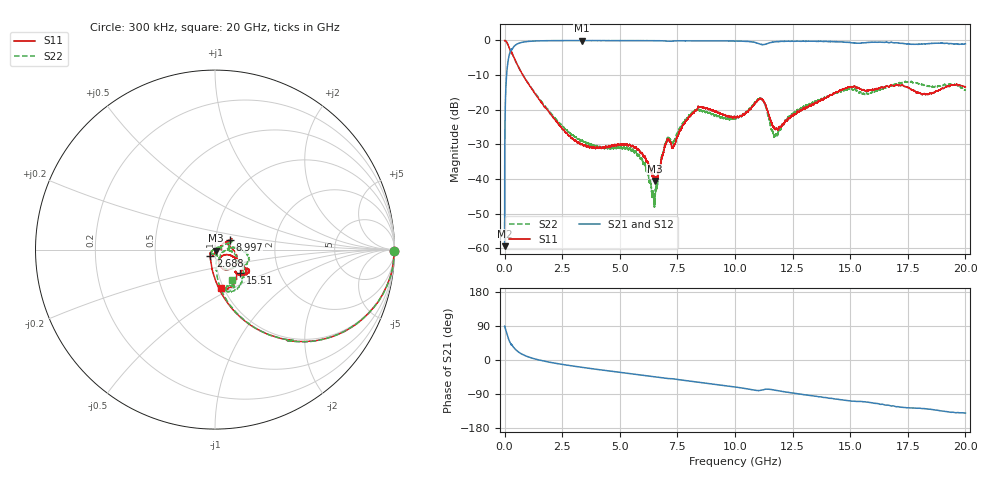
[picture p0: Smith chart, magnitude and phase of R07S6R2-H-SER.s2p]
!{R07S6R2}
!Johanson Technology Inc.
!www.johansontechnology.com
!Test Board Conditions:
!Substrate Type  RO4350B
!Substrate Thickness  10 mil
!Substrate Dk  3.66
!TL Type: GCPW
!TL Trace Width  21 mil
!TL Gap  20 mil
!Electrode orientation  Horizontal
!DUT TOPOLOGY	SERIES
!Mounting Pad LxW  16x21 mil
! Created Sat Feb  6 11:37:33 2021
# hz S ma R 50
! 2 Port Network Data from SP1.SP block
! freq  magS11  angS11  magS21  angS21  magS12  angS12  magS22  angS22
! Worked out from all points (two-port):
!   20001 points, 300 kHz to 20 GHz, reference 50 ohm
!   highest |S21| = -0.03 dB at 3.357 GHz (marker M1); lowest = -59.4 dB at 300 kHz (marker M2)
!   |S21| within 3 dB of the highest: 257.6 MHz to end of sweep
!   lowest |S11| = -40.5 dB at 6.525 GHz (marker M3), VSWR 1.02, Z = 50.7 - j0.674 ohm
!   |S11| at or under -10 dB: 794.4 MHz to end of sweep
!   |S22| runs from -48.2 to 0.0 dB; largest |S21 - S12| = 0.012
!   S11 on the Smith chart (normalised r, x): 300 kHz: open; 2.688 GHz: 0.95, -0.07; 8.997 GHz: 1.17, +0.13; 15.51 GHz: 1.28, -0.35; 20 GHz: 0.97, -0.43
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300000  0.9982 -0.4  0.001074 89.1  0.001152 93.4  0.9994 -0.4
1.093e8  0.919 -23.7  0.3903 66.6  0.3907 66.6  0.919 -23.6
2.833e8  0.6659 -49.9  0.7374 40.8  0.7376 40.7  0.6686 -49.8
9.053e8  0.2741 -79.2  0.9581 11.1  0.9587 11.1  0.2772 -77.8
2.6883e9  0.04622 -125.2  0.9949 -13.3  0.9957 -13.4  0.05084 -77.8
3.3343e9  0.0319 -144.2  0.9953 -19.1  0.996 -19.1  0.03585 -69.2
3.3573e9  0.03183 -144.9  0.9968 -19.3  0.9959 -19.3  0.036 -69.0
5.6323e9  0.0282 -109.2  0.9925 -37.5  0.9935 -37.5  0.02409 -141.8
6.5253e9  0.009416 -44.9  0.9919 -44.6  0.9918 -44.6  0.005167 92.2
6.6673e9  0.01203 -5.2  0.9913 -45.7  0.9913 -45.7  0.01141 53.4
7.0653e9  0.03683 9.1  0.9764 -49.0  0.9767 -49.0  0.03949 16.8
7.3393e9  0.03053 19.7  0.982 -50.0  0.9828 -49.9  0.03534 17.6
8.3043e9  0.09767 32.0  0.9851 -57.7  0.9866 -57.8  0.09887 26.4
8.9973e9  0.09773 33.4  0.9839 -63.0  0.986 -63.0  0.08655 18.1
1.00003e10  0.07869 23.7  0.9811 -71.2  0.9827 -71.3  0.07396 -1.4
1.11343e10  0.1441 -42.8  0.8774 -79.7  0.8767 -79.7  0.147 -42.5
1.17663e10  0.05275 -51.4  0.9583 -80.0  0.9587 -80.0  0.04403 -31.2
1.33343e10  0.1175 -21.6  0.9731 -94.2  0.9729 -94.3  0.1245 2.8
1.55093e10  0.1927 -42.8  0.9233 -109.8  0.9198 -109.7  0.17 -28.2
1.66673e10  0.2152 -30.6  0.9296 -119.4  0.9348 -119.9  0.2149 -42.4
1.83233e10  0.1679 -47.4  0.8961 -129.0  0.8972 -129.1  0.223 -73.8
2e10  0.2142 -81.1  0.8945 -139.9  0.888 -139.9  0.192 -60.8
